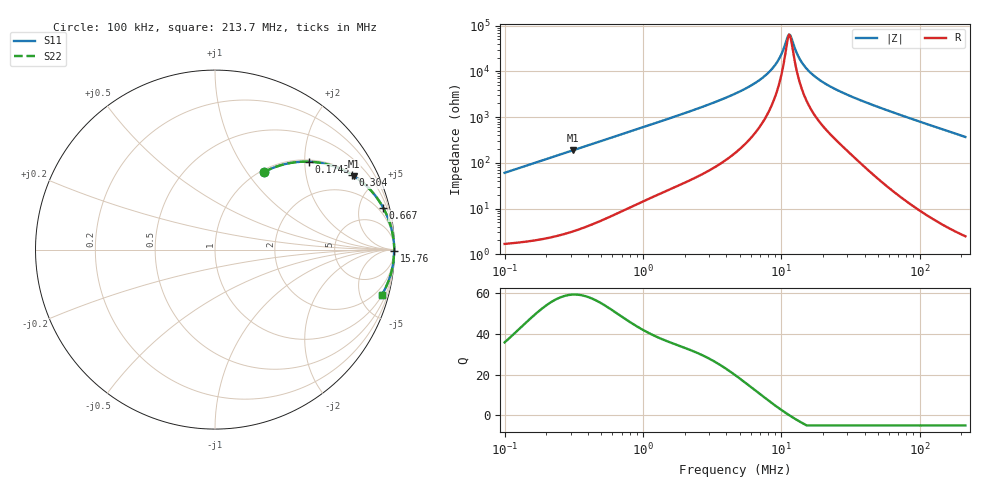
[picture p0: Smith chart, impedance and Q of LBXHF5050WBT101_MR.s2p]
! LBXHF5050WBT101_MR  S-PARAMETER MODEL  ( General Type )
! Model Generated by TAIYO YUDEN Corporation (http://www.ty-top.com)
! Version 1.0
! TAIYO YUDEN Control No. 210719NI43SB-FBB
! Copyright(c) 2021 TAIYO YUDEN CO.,LTD. All Rights Reserved.
! Product Description (link to TY-COMPAS)
! https://ds.yuden.co.jp/TYCOMPAS/or/detail?pn=LBXHF5050WBT101MMR&u=M
! Products Name : Inductors
! Characteristics :
!  Inductance : 100 uH , SRF(min) : 8.0 MHz , DC Resistance(max) : 1.02 Ohm
!  Rated Current : Saturation :500 mA , Temp Rise : 420 mA
!  Case Size : 5.0 x 5.0 / 0.197 x 0.197 [mm/inch] , Thickness : 2.2 / 0.087 [mm/inch]
!  (Conditions: Temperature = 25 degC , DC Bias Current/Voltage = 0A / 0V)
! External Node Assignments :
!  1  o---GGG---o  2
! GND o---------o GND
! Frequency Range : 0.1MHz  -  213.673535MHz  [ 402 STEP ]
# MHz S RI R 50
! Freq[MHz].  S11 Real  S11 Imag  S21 Real  S21 Imag  S12 Real  S12 Imag  S22 Real  S22 Imag
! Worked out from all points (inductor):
!   401 points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, 100 kHz to 213.7 MHz, reference 50 ohm
!   read as one part in series: L = 95.9 uH near 103.9 kHz
!   highest Q = 59.4 at 309.8 kHz (marker M1), where L = 95.7 uH
!   self-resonance near 11.38 MHz
!   S11 on the Smith chart (normalised r, x): 100 kHz: 1.03, +1.21; 174.3 kHz: 1.04, +2.10; 304 kHz: 1.06, +3.66; 667 kHz: 1.16, +8.01; 15.76 MHz: open; 213.7 MHz: 1.05, -7.35
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0.1  0.2728 0.4317  0.7272 -0.4317  0.7272 -0.4317  0.2728 0.4317
0.174344  0.5239 0.4897  0.4761 -0.4897  0.4761 -0.4897  0.5239 0.4897
0.303958  0.766 0.4151  0.234 -0.4151  0.234 -0.4151  0.766 0.4151
0.309841  0.7726 0.4108  0.2274 -0.4108  0.2274 -0.4108  0.7726 0.4108
0.361188  0.821 0.375  0.179 -0.375  0.179 -0.375  0.821 0.375
0.666981  0.9372 0.2328  0.0628 -0.2328  0.0628 -0.2328  0.9372 0.2328
1.304567  0.9809 0.1246  0.0191 -0.1246  0.0191 -0.1246  0.9809 0.1246
4.71194  0.9976 0.0299  0.00244 -0.0299  0.00244 -0.0299  0.9976 0.0299
6.653322  0.9983 0.0169  0.00174 -0.0169  0.00174 -0.0169  0.9983 0.0169
8.373963  0.9985 0.00937  0.00155 -0.00937  0.00155 -0.00937  0.9985 0.00937
9.576387  0.9985 0.00525  0.00152 -0.00525  0.00152 -0.00525  0.9985 0.00525
10.1432  0.9985 0.00353  0.00152 -0.00353  0.00152 -0.00353  0.9985 0.00353
10.95147  0.9985 0.00125  0.00154 -0.00125  0.00154 -0.00125  0.9985 0.00125
11.37945  0.9984 0.000113  0.00155 -0.000113  0.00155 -0.000113  0.9984 0.000113
11.82415  0.9984 -0.00102  0.00157 0.00102  0.00157 0.00102  0.9984 -0.00102
13.52199  0.9983 -0.00499  0.00167 0.00499  0.00167 0.00499  0.9983 -0.00499
15.76288  0.9982 -0.0096  0.00183 0.0096  0.00183 0.0096  0.9982 -0.0096
16.69585  0.9981 -0.0114  0.00191 0.0114  0.00191 0.0114  0.9981 -0.0114
20.22332  0.9978 -0.0175  0.0022 0.0175  0.0022 0.0175  0.9978 -0.0175
25.94593  0.9974 -0.0264  0.00265 0.0264  0.00265 0.0264  0.9974 -0.0264
60.30341  0.9931 -0.0732  0.00691 0.0732  0.00691 0.0732  0.9931 -0.0732
213.6735  0.9296 -0.2525  0.0704 0.2525  0.0704 0.2525  0.9296 -0.2525
